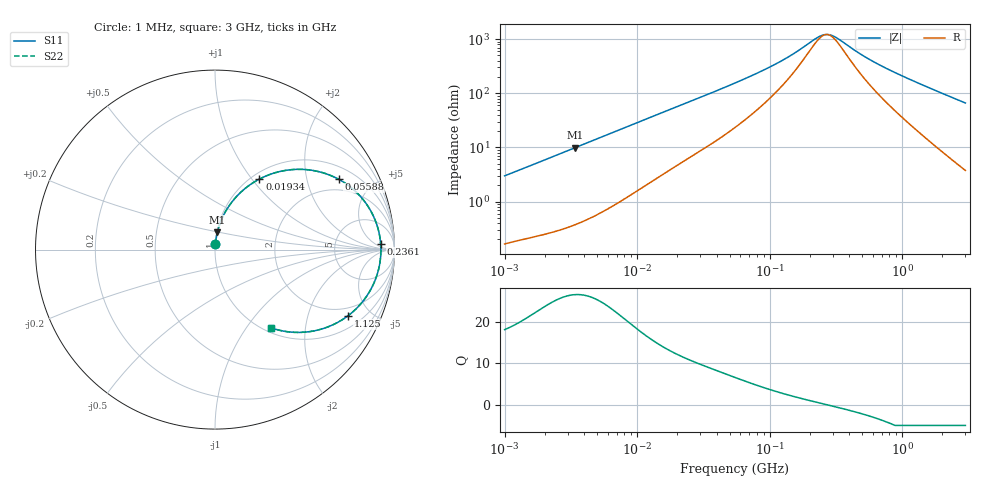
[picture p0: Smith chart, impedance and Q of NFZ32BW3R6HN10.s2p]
! NFZ32BW3R6HN10
# Hz S RI R 50
!Freq.(Hz) S11(Real) S11(Imag) S21(Real) S21(Imag) S12(Real) S12(Imag) S22(Real) S22(Imag)
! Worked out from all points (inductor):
!   401 points, 1 MHz to 3 GHz, reference 50 ohm
!   read as one part in series: L = 470 nH near 1.041 MHz
!   highest Q = 26.5 at 3.39 MHz (marker M1), where L = 462 nH
!   self-resonance near 269.5 MHz
!   S11 on the Smith chart (normalised r, x): 1 MHz: 1.00, +0.06; 19.34 MHz: 1.09, +1.09; 55.88 MHz: 1.48, +3.13; 236.1 MHz: 21, +9; 1.125 GHz: 1.55, -3.63; 3 GHz: 1.08, -1.32
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1000000  0.00253 0.0297  0.9975 -0.0297  0.9975 -0.0297  0.00253 0.0297
3390478  0.0132 0.0968  0.9868 -0.0968  0.9868 -0.0968  0.0132 0.0968
3823119  0.0162 0.1086  0.9838 -0.1086  0.9838 -0.1086  0.0162 0.1086
8179831  0.0621 0.2181  0.9379 -0.2181  0.9379 -0.2181  0.0621 0.2181
1.461624e7  0.164 0.3375  0.836 -0.3375  0.836 -0.3375  0.164 0.3375
1.934349e7  0.2474 0.3929  0.7526 -0.3929  0.7526 -0.3929  0.2474 0.3929
3.320783e7  0.4672 0.4474  0.5328 -0.4474  0.5328 -0.4474  0.4672 0.4474
5.477226e7  0.681 0.3961  0.319 -0.3961  0.319 -0.3961  0.681 0.3961
5.587962e7  0.6884 0.3922  0.3116 -0.3922  0.3116 -0.3922  0.6884 0.3922
8.011685e7  0.8008 0.3065  0.1992 -0.3065  0.1992 -0.3065  0.8008 0.3065
1.148668e8  0.8709 0.21  0.1291 -0.21  0.1291 -0.21  0.8709 0.21
1.520175e8  0.9021 0.1373  0.0979 -0.1373  0.0979 -0.1373  0.9021 0.1373
2.094008e8  0.9202 0.0592  0.0798 -0.0592  0.0798 -0.0592  0.9202 0.0592
2.361213e8  0.9232 0.0309  0.0768 -0.0309  0.0768 -0.0309  0.9232 0.0309
2.716345e8  0.9244 -0.00188  0.0756 0.00188  0.0756 0.00188  0.9244 -0.00188
3.062963e8  0.9235 -0.03  0.0765 0.03  0.0765 0.03  0.9235 -0.03
5.154121e8  0.8971 -0.1576  0.1029 0.1576  0.1029 0.1576  0.8971 -0.1576
8.005644e8  0.8325 -0.2771  0.1675 0.2771  0.1675 0.2771  0.8325 -0.2771
1.125055e9  0.7412 -0.3685  0.2588 0.3685  0.2588 0.3685  0.7412 -0.3685
1.855641e9  0.5358 -0.4558  0.4642 0.4558  0.4642 0.4558  0.5358 -0.4558
2.312676e9  0.4313 -0.4604  0.5687 0.4604  0.5687 0.4604  0.4313 -0.4604
3e9  0.3141 -0.4366  0.6859 0.4366  0.6859 0.4366  0.3141 -0.4366
